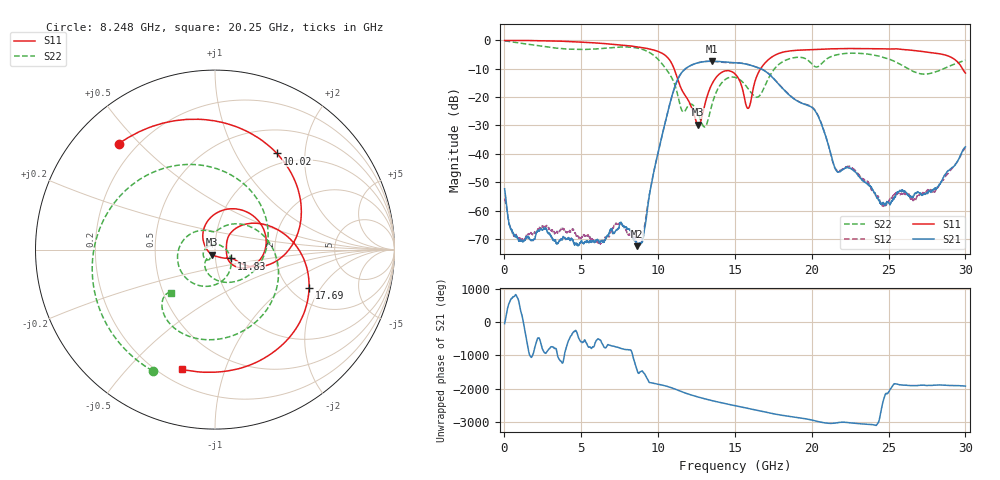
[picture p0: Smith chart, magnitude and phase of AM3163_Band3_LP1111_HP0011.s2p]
!Agilent Technologies,E8364B,MY43040894,A.07.50.67
!Agilent E8364B: A.07.50.67
!Date: Thursday, August 20, 2020 12:15:22
!Correction: S11(Full 2 Port(1,2))
!S21(Full 2 Port(1,2))
!S12(Full 2 Port(1,2))
!S22(Full 2 Port(1,2))
!S2P File: Measurements: S11, S21, S12, S22:
# Hz S  dB  R 50
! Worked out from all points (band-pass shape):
!   3201 points, 10 MHz to 30 GHz, reference 50 ohm
!   highest |S21| = -7.31 dB at 13.52 GHz (marker M1); lowest = -72.6 dB at 8.651 GHz (marker M2)
!   |S21| within 3 dB of the highest: 11.71 GHz to 16.81 GHz (5.099 GHz wide, 35.8 % of centre)
!   lowest |S11| = -29.7 dB at 12.62 GHz (marker M3), VSWR 1.07, Z = 48.4 - j2.81 ohm
!   |S11| at or under -10 dB: 11.04 GHz to 16.67 GHz (5.626 GHz wide, 40.6 % of centre); 29.81 GHz to end of sweep
!   |S22| runs from -30.5 to -0.1 dB; largest |S21 - S12| = 0.013
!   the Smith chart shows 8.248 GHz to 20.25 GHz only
!   S11 on the Smith chart (normalised r, x): 8.248 GHz: 0.13, +0.44; 10.02 GHz: 0.83, +1.50; 11.83 GHz: 1.19, -0.12; 17.69 GHz: 2.49, -1.57; 20.25 GHz: 0.28, -0.73
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1e7  -0.02 -1.9  -52.32 -54.3  -55.79 -62.0  -0.14 -4.9
1.247088e9  -0.00 -34.1  -70.54 -51.8  -70.34 109.6  -1.12 -82.6
2.652869e9  -0.11 -72.3  -66.51 142.8  -65.63 9.8  -2.22 -162.8
5.014581e9  -0.60 -134.8  -70.59 120.2  -69.39 10.9  -3.19 72.1
6.589056e9  -1.13 -177.3  -69.85 -58.5  -69.79 124.1  -2.69 -16.4
8.247878e9  -1.97 132.3  -67.57 -144.2  -68.58 47.1  -2.39 -117.2
8.650869e9  -2.24 118.1  -72.57 -45.8  -71.86 -146.8  -2.68 -144.7
1.000979e10  -3.90 57.7  -39.20 -69.1  -39.30 -69.6  -6.71 93.3
1.001916e10  -3.92 57.2  -38.97 -70.1  -39.07 -70.5  -6.76 92.1
1.089075e10  -8.16 -3.8  -19.79 -179.1  -19.91 -178.9  -13.21 -51.4
1.182793e10  -19.92 -29.1  -9.79 16.3  -9.82 16.7  -24.14 -119.3
1.261517e10  -29.69 -117.9  -7.85 -95.7  -7.83 -95.3  -25.92 170.9
1.352424e10  -15.18 100.2  -7.31 155.9  -7.38 155.3  -22.26 -13.4
1.5005e10  -11.79 -12.5  -7.83 6.8  -7.90 8.5  -13.03 -152.2
1.586721e10  -23.94 4.6  -8.53 -76.6  -8.46 -76.0  -17.06 132.0
1.769473e10  -4.94 -22.3  -14.52 106.9  -14.41 107.4  -9.26 -7.3
2.000958e10  -3.25 -99.3  -23.63 -65.7  -23.45 -65.3  -8.32 -137.4
2.025325e10  -3.20 -105.2  -25.11 -92.8  -24.93 -92.8  -9.32 -135.2
2.16028e10  -2.92 -136.9  -45.94 -149.0  -45.68 -146.7  -5.08 -160.3
2.500479e10  -3.00 144.7  -57.16 56.2  -56.69 -154.4  -6.55 67.6
2.740399e10  -4.03 77.4  -54.00 -104.6  -53.34 -105.4  -11.88 -88.0
3e10  -11.49 -28.8  -37.54 -125.6  -37.92 -125.1  -6.97 130.3
